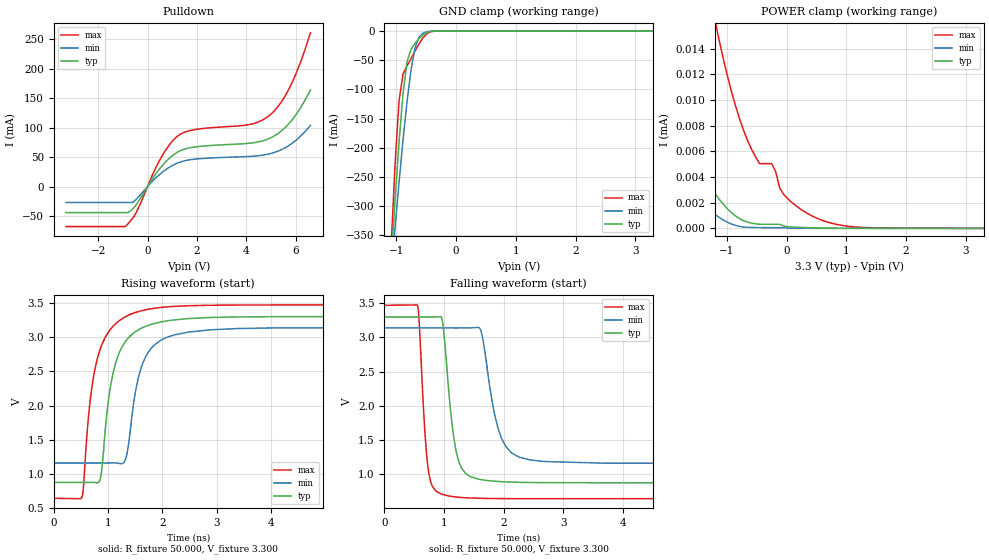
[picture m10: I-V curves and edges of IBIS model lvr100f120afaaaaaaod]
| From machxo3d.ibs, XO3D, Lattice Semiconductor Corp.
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|   Model lvr100f120afaaaaaaod
[Model] lvr100f120afaaaaaaod
Model_type I/O_open_drain
Polarity   Non-Inverting
Enable   Active-Low
Vinl =  0.350V
Vinh =  0.650V
Vmeas =  0.500V
Cref =  0.0F
Rref = 10.00k
Vref = 1.00V
C_comp   4.200pF   3.800pF   7.500pF
[Temperature Range]   25.000   0.105k   -40.000
[Voltage Range]   3.300V   3.140V   3.470V
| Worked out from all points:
|   slope of the pulldown table from 0 to 0.495 V, typ, clamps not added: 16.2 ohm
|   GND clamp passes 1 mA (typ) near -0.43 V on its own axis
|   rising waveform, R_fixture 50.000, V_fixture 3.300: 20-80 % time 311ps typ, 318ps min, 315ps max; typ from 0.878 V to 3.3 V
|   falling waveform, R_fixture 50.000, V_fixture 3.300: 20-80 % time 176ps typ, 260ps min, 115ps max; typ from 3.3 V to 0.878 V
[Pulldown]
|Voltage   I(typ)   I(min)   I(max)
-3.3V     -43.98mA   -26.85mA   -67.81mA
-900mV    -43.98mA   -26.85mA   -67.81mA
-500mV    -33.06mA   -23.42mA   -47.39mA
600mV     35.86mA    24.47mA    52.84mA
1.2V      58.2mA     39.81mA    85.22mA
1.9V      67.18mA    46.57mA    96.69mA
4.2V      73.98mA    51.49mA    106.1mA
4.9V      81.14mA    55.32mA    119.6mA
5.4V      93.79mA    62.3mA     142.5mA
5.8V      110.5mA    71.89mA    171.7mA
6.2V      134mA      85.76mA    211.4mA
6.6V      164mA      103.9mA    261.1mA
[GND_clamp]
|Voltage   I(typ)   I(min)   I(max)
-3.3V     -4.507A    -3.482A    -6.263A
-1.089V   -398.4mA   -420.6mA   -374.7mA
-1.022V   -290.7mA   -338.6mA   -230.6mA
-955mV    -191.4mA   -260.2mA   -120.1mA
-888mV    -107.5mA   -187mA     -73.69mA
-821mV    -53mA      -121.4mA   -59.83mA
-754mV    -31.41mA   -66.95mA   -47.44mA
-687mV    -21.17mA   -28.83mA   -34.23mA
-620mV    -13.21mA   -10.24mA   -21.98mA
-553mV    -6.877mA   -3.592mA   -11.71mA
-352mV    -122.8uA   -54.62uA   -209.3uA
3.3V      0A         0A         0A
[POWER_clamp]
|Voltage   I(typ)   I(min)   I(max)
-3.3V     530uA      347.3uA    956.2uA
-2.663V   63.57uA    15.44uA    254.2uA
-2.529V   27.42uA    10.98uA    148.7uA
-2.328V   15.78uA    8.532uA    64.82uA
-1.725V   7.398uA    3.713uA    31uA
-1.189V   2.659uA    1.053uA    15.99uA
-988mV    1.516uA    474.5nA    11.83uA
-519mV    357.5nA    63.28nA    5.567uA
-251mV    319nA      55.54nA    5.047uA
-50mV     187.6nA    55.54nA    2.655uA
352mV     56.19nA    7.349nA    1.154uA
3.3V      0A         0A         0A
[Ramp]
| variable   typ   min   max
dV/dt_r   1.453/0.314n   1.187/0.316n   1.694/0.315n
dV/dt_f   1.453/0.175n   1.187/0.259n   1.694/0.114n
R_load = 50.000
[Rising Waveform]
R_fixture= 50.000
V_fixture= 3.300
V_fixture_min= 3.140
V_fixture_max= 3.470
|time   V(typ)   V(min)   V(max)
0s        878.1mV    1.161V     645.8mV
527ps     878.1mV    1.161V     681.6mV
674ps     879mV      1.161V     2.1V
842ps     898.9mV    1.161V     2.794V
1.06ns    2.35V      1.163V     3.128V
1.296ns   2.909V     1.175V     3.286V
1.548ns   3.1V       2.376V     3.369V
1.742ns   3.172V     2.781V     3.407V
3.389ns   3.295V     3.125V     3.468V
20ns      3.3V       3.14V      3.47V
[Falling Waveform]
R_fixture= 50.000
V_fixture= 3.300
V_fixture_min= 3.140
V_fixture_max= 3.470
|time   V(typ)   V(min)   V(max)
0s        3.3V       3.14V      3.47V
558ps     3.3V       3.14V      3.465V
745ps     3.298V     3.14V      1.021V
970ps     3.256V     3.14V      708.8mV
1.106ns   1.968V     3.139V     681.6mV
1.359ns   1.016V     3.14V      659.3mV
1.615ns   924.1mV    3.108V     650.9mV
1.966ns   894.1mV    1.525V     647.3mV
2.451ns   882.2mV    1.211V     646.2mV
20ns      878.1mV    1.161V     645.8mV
